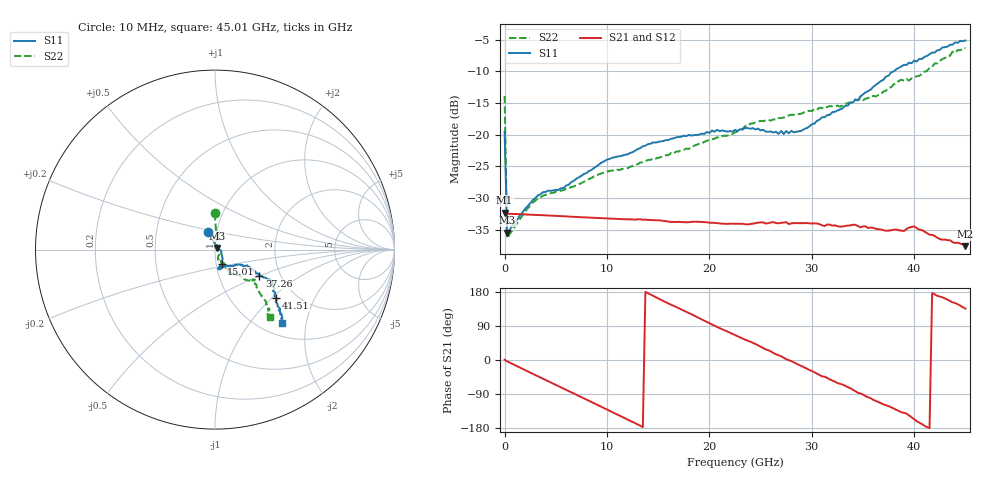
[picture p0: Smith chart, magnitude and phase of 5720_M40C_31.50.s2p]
! Device:  ADRF5720
! Description: 0.5dB LSB GaAs MMIC 6-bit Digital Attenuator
! Frequency:  0.000009 -  40 GHz
! Ports:
!	RF1	= Port 1
!	RF2	= Port 2
! Vdd:  3.3 Volt
! Vss:  -3.3 Volt
! Control:  0/3.3 Volt
! State:  31.50 dB attenuation
! Data:  The device was measured using G-S-G Probes on a matrix board.
!  Data was collected using an calibrated 4 port network analyzer.
!  The reference plane for this measurement is at the launchers.
! Note:  Analog Devices supplies this data as a sample of measured data
!  for this product.  Your particular data for this product may vary.
!  Data was taken at -40 degrees C.
!  Analog Devices reserves the right to change this data at anytime.
# GHZ S DB R 45.0
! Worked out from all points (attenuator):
!   181 points, 10 MHz to 45.01 GHz, reference 45 ohm
!   highest |S21| = -32.30 dB at 10 MHz (marker M1); lowest = -37.6 dB at 45.01 GHz (marker M2)
!   lowest |S11| = -35.5 dB at 260 MHz (marker M3), VSWR 1.03, Z = 46.3 + j0.884 ohm
!   |S11| at or under -10 dB: start of sweep to 38.01 GHz
!   |S22| runs from -36.4 to -6.3 dB; largest |S21 - S12| = 0.00018
!   S11 on the Smith chart (normalised r, x): 10 MHz: 0.91, +0.18; 15.01 GHz: 1.06, -0.17; 37.26 GHz: 1.56, -0.50; 41.51 GHz: 1.60, -1.06; 45.01 GHz: 1.23, -1.46
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0.01  -19.53 112.3  -32.30 0.6  -32.31 0.4  -13.89 90.4
0.26  -35.50 34.7  -32.49 -3.6  -32.50 -3.6  -36.38 33.2
3.26  -29.59 -8.9  -32.69 -43.0  -32.71 -43.0  -30.05 -32.0
5.76  -28.43 -25.0  -32.88 -75.4  -32.90 -75.4  -28.79 -52.0
7.76  -26.19 -39.2  -33.05 -101.3  -33.06 -101.3  -27.42 -65.9
10.01  -23.92 -48.2  -33.23 -130.7  -33.25 -130.7  -25.83 -70.0
15.01  -21.15 -65.5  -33.53 162.7  -33.54 162.7  -23.64 -67.2
15.26  -21.04 -66.5  -33.55 159.1  -33.57 159.0  -23.55 -67.4
20.26  -19.34 -77.9  -33.91 93.8  -33.93 93.7  -20.74 -58.8
22.76  -19.40 -80.2  -34.07 62.8  -34.10 62.8  -19.51 -59.2
24.01  -19.06 -75.3  -34.11 48.2  -34.13 48.1  -18.25 -58.1
27.26  -19.89 -65.7  -33.88 6.2  -33.89 6.1  -17.28 -56.1
30.26  -18.24 -47.2  -34.00 -32.3  -34.03 -32.3  -15.96 -57.3
32.76  -16.02 -31.4  -34.53 -62.9  -34.56 -62.9  -15.56 -53.2
34.76  -13.97 -26.0  -34.63 -88.3  -34.66 -88.3  -14.25 -49.3
37.26  -10.82 -30.6  -35.18 -119.3  -35.19 -119.5  -13.04 -46.1
37.76  -10.16 -30.1  -35.09 -124.7  -35.09 -124.7  -12.50 -44.8
38.76  -9.22 -28.6  -35.16 -137.9  -35.15 -137.9  -11.30 -40.4
40.01  -8.29 -31.7  -34.48 -156.2  -34.49 -156.1  -11.05 -38.8
41.51  -7.27 -38.4  -35.80 -179.4  -35.78 -179.5  -9.43 -43.5
43.76  -5.78 -44.0  -36.98 152.3  -36.98 152.2  -6.88 -47.7
45.01  -5.11 -47.7  -37.61 135.5  -37.61 135.8  -6.30 -51.0
